DATA_BLOCK "DatiPerOP"
TITLE =
VERSION : 0.1


  STRUCT
   PressureTank_S1 : REAL ;	//PRESSURE INDICATOR 004600VA002A (0-16 bar) S1 - EW30 - 6005004600PT015
   PressureTank_S2 : REAL ;	//PRESSURE INDICATOR 004600VA002B (0-16 bar) S2 - EW32 - 6005004600PT016
   PressureTank_S3 : REAL ;	//PRESSURE INDICATOR 004600VA003 (0-16 bar) S3 - EW34 - 6005004600PT017
   PressureTank_S4 : REAL ;	//PRESSURE INDICATOR
   TemperatureTank_S1 : REAL ;	//TEMPERATURE INDICATOR 004600VA002A (0-60 °C) S1 - EW40 - 6005004600TT002
   TemperatureTank_S2 : REAL ;	//TEMPERATURE INDICATOR 004600VA002B (0-60 °C) S2 - EW42 - 6005004600TT003
   TemperatureTank_S3 : REAL ;	//TEMPERATURE INDICATOR 004600VA003 ((0-60 °C) S3 - EW44 - 6005004600TT004
   TemperatureTank_S4 : REAL ;	//TEMPERATURE INDICATOR
   HumidutyLine : REAL ;	//HUMIDUTY INDICATOR - EW52 - 6005004600AT001
   PressureLine : REAL ;	//PRESSURE INDICATOR LINE 004600IA046-2"-A55-N  (0-16 bar)-EW50 - 6005004600PT014
   FlowLine : REAL ;	//FLOW INDICATOR - EW54 - 6005004600FT001
   TemperatureComp_A : REAL ;	//TEMPERATURE INDICATOR COMPRESSOR A - 6005004600TT010A
   PressureComp_A : REAL ;	//PRESSURE INDICATOR COMPRESSOR A - 6005004600PT011A
   TemperatureComp_B : REAL ;	//TEMPERATURE INDICATOR COMPRESSOR B -6005004600TT010B
   PressureComp_B : REAL ;	//PRESSURE INDICATOR COMPRESSOR B - 6005004600PT011B
   TemperatureComp_C : REAL ;	//TEMPERATURE INDICATOR COMPRESSOR C - 6005004600TT010B
   PressureComp_C : REAL ;	//PRESSURE INDICATOR COMPRESSOR C -6005004600PT011B

T6005004600UY007 : INT ;	//CLS VALVE UV007 FOR LOW PRES.(6barg)-6005004600UY007
T6005004600ZLH007 : INT ;	//VALVE UV007 OPEN - 6005004600ZLH007
T6005004600ZLL007 : INT ;	//VALVE UV007 CLOSE - 6005004600ZLL007
T6005004600UL101 : INT ;	//COLUMN A ON LINE  - 6005004600UL101
T6005004600UL102 : INT ;	//COLUMN A REGENERETING  - 6005004600UL102
T6005004600UL108 : INT ;	//COLUMN A RE-PRESSURING - 6005004600UL108
T6005004600UL109 : INT ;	//COLUMN A STAND BY - 6005004600UL109
T6005004600UL115 : INT ;	//COLUMN B ON LINE  - 6005004600UL115
T6005004600UL116 : INT ;	//COLUMN B REGENERETING  - 6005004600UL116
T6005004600UL122 : INT ;	//COLUMN B RE-PRESSURING - 6005004600UL122
T6005004600UL123 : INT ;	//COLUMN B STAND BY - 6005004600UL123
T6005004600UA130 : INT ;	//DEW POINT ALARM - 6005004600UA130
T6005004600UA136 : INT ;	//SENSOR ERROR - 6005004600UA136
T6005004600UL137 : INT ;	//SERVICE INTERVAL - 6005004600UL137
T6005004600UL111 : INT ;	//FAULT RELAY ACTIVE - 6005004600UL111
T6005004600UL201 : INT ;	//COLUMN A ON LINE  - 6005004600UL201
T6005004600UL202 : INT ;	//COLUMN A REGENERETING  - 6005004600UL202
T6005004600UL208 : INT ;	//COLUMN A RE-PRESSURING - 6005004600UL208
T6005004600UL209 : INT ;	//COLUMN A STAND BY - 6005004600UL209
T6005004600UL215 : INT ;	//COLUMN B ON LINE  - 6005004600UL215
T6005004600UL216 : INT ;	//COLUMN B REGENERETING  - 6005004600UL216
T6005004600UL222 : INT ;	//COLUMN B REPRESSURING - 6005004600UL222
T6005004600UL223 : INT ;	//COLUMN B STAND BY - 6005004600UL223
T6005004600UA230 : INT ;	//DEW POINT ALARM - 6005004600UA230
T6005004600UA236 : INT ;	//SENSOR ERROR - 6005004600UA236
T6005004600UL237 : INT ;	//SERVICE INTERVAL - 6005004600UL237
T6005004600UL211 : INT ;	//FAULT RELAY ACTIVE - 6005004600UL211
T6005004600UL301 : INT ;	//COLUMN A ON LINE  - 6005004600UL301
T6005004600UL302 : INT ;	//COLUMN A REGENERETING  - 6005004600UL302
T6005004600UL308 : INT ;	//COLUMN A RE-PRESSURING - 6005004600UL308
T6005004600UL309 : INT ;	//COLUMN A STAND BY - 6005004600UL309
T6005004600UL315 : INT ;	//COLUMN B ON LINE  - 6005004600UL315
T6005004600UL316 : INT ;	//COLUMN B REGENERETING  - 6005004600UL316
T6005004600UL322 : INT ;	//COLUMN B REPRESSURING - 6005004600UL322
T6005004600UL323 : INT ;	//COLUMN B STAND BY - 6005004600UL323
T6005004600UA330 : INT ;	//DEW POINT ALARM - 6005004600UA330
T6005004600UA336 : INT ;	//SENSOR ERROR - 6005004600UA336
T6005004600UL337 : INT ;	//SERVICE INTERVAL - 6005004600UL337
T6005004600UL311 : INT ;	//FAULT RELAY ACTIVE - 6005004600UL311
T6005004600UL001A : INT ;	//RUN / STOP COMPRESSOR A - 6005004600UL001A
T6005004600UL002A : INT ;	//LOAD / UNLOAD COMPRESSOR A  - 6005004600UL002A
T6005004600UA003A : INT ;	//GENERAL WARNING COMPRESSOR A  - 6005004600UA003A
T6005004600UA012A : INT ;	//SENSOR ERROR COMPRESSOR A  - 6005004600UA012A
T6005004600UL001B : INT ;	//RUN / STOP COMPRESSOR B - 6005004600UL001B
T6005004600UL002B : INT ;	//LOAD / UNLOAD COMPRESSOR B - 6005004600UL002B
T6005004600UA003B : INT ;	//GENERAL WARNING COMPRESSOR B - 6005004600UA003B
T6005004600UA012B : INT ;	//SENSOR ERROR COMPRESSOR B - 6005004600UA012B
T6005004600UL001C : INT ;	//RUN / STOP COMPRESSOR C - 6005004600UL001C
T6005004600UL002C : INT ;	//LOAD / UNLOAD COMPRESSOR C - 6005004600UL002C
T6005004600UA003C : INT ;	//GENERAL WARNING COMPRESSOR C - 6005004600UA003C
T6005004600UA012C : INT ;	//SENSOR ERROR COMPRESSOR C - 6005004600UA012C

  END_STRUCT ;
BEGIN
   PressureTank_S1 := 0.000000e+000;
   PressureTank_S2 := 0.000000e+000;
   PressureTank_S3 := 0.000000e+000;
   PressureTank_S4 := 0.000000e+000;
   TemperatureTank_S1 := 0.000000e+000;
   TemperatureTank_S2 := 0.000000e+000;
   TemperatureTank_S3 := 0.000000e+000;
   TemperatureTank_S4 := 0.000000e+000;
   HumidutyLine := 0.000000e+000;
   PressureLine := 0.000000e+000;
   FlowLine := 0.000000e+000;
   TemperatureComp_A := 0.000000e+000;
   PressureComp_A := 0.000000e+000;
   TemperatureComp_B := 0.000000e+000;
   PressureComp_B := 0.000000e+000;
   TemperatureComp_C := 0.000000e+000;
   PressureComp_C := 0.000000e+000;
   T6005004600UY007 : =0;
T6005004600ZLH007 : =0;
T6005004600ZLL007 : =0;
T6005004600UL101 : =0;
T6005004600UL102 : =0;
T6005004600UL108 : =0;
T6005004600UL109 : =0;
T6005004600UL115 : =0;
T6005004600UL116 : =0;
T6005004600UL122 : =0;
T6005004600UL123 : =0;
T6005004600UA130 : =0;
T6005004600UA136 : =0;
T6005004600UL137 : =0;
T6005004600UL111 : =0;
T6005004600UL201 : =0;
T6005004600UL202 : =0;
T6005004600UL208 : =0;
T6005004600UL209 : =0;
T6005004600UL215 : =0;
T6005004600UL216 : =0;
T6005004600UL222 : =0;
T6005004600UL223 : =0;
T6005004600UA230 : =0;
T6005004600UA236 : =0;
T6005004600UL237 : =0;
T6005004600UL211 : =0;
T6005004600UL301 : =0;
T6005004600UL302 : =0;
T6005004600UL308 : =0;
T6005004600UL309 : =0;
T6005004600UL315 : =0;
T6005004600UL316 : =0;
T6005004600UL322 : =0;
T6005004600UL323 : =0;
T6005004600UA330 : =0;
T6005004600UA336 : =0;
T6005004600UL337 : =0;
T6005004600UL311 : =0;
T6005004600UL001A : =0;
T6005004600UL002A : =0;
T6005004600UA003A : =0;
T6005004600UA012A : =0;
T6005004600UL001B : =0;
T6005004600UL002B : =0;
T6005004600UA003B : =0;
T6005004600UA012B : =0;
T6005004600UL001C : =0;
T6005004600UL002C : =0;
T6005004600UA003C : =0;
T6005004600UA012C : =0;

END_DATA_BLOCK

